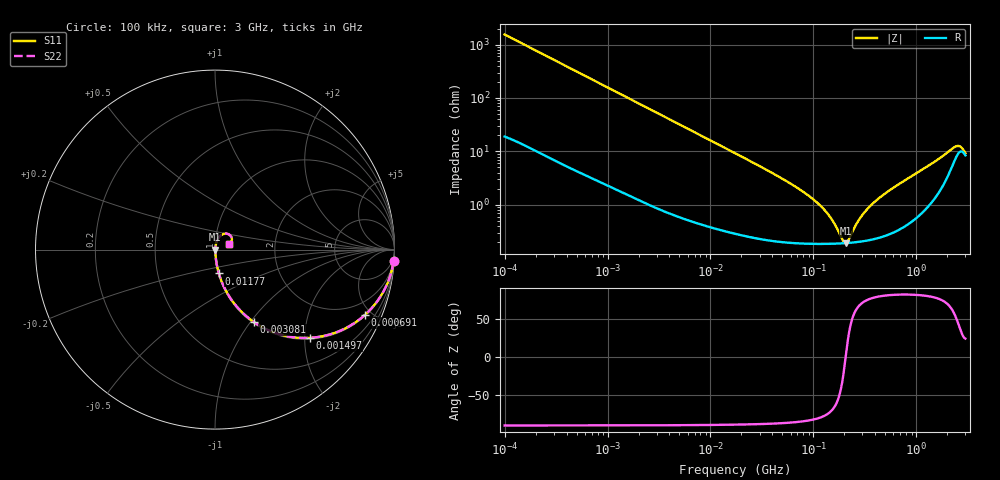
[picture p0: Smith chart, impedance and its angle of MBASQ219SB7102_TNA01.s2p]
! MBASQ219SB7102_TNA01  S-PARAMETER MODEL  ( Standard Model )
! Model Generated by TAIYO YUDEN Corporation (http://www.ty-top.com)
! Version 1.0
! TAIYO YUDEN Control No. 220601
! Copyright(c) 2013 TAIYO YUDEN CO.,LTD. All Rights Reserved.
! Product Description (link to TY-COMPAS)
! https://ds.yuden.co.jp/TYCOMPAS/or/detail?pn=MBASQ219SB7102KTNA01&u=M
! Products Name : Multilayer Ceramic Capacitors
! Characteristics :
!  Capacitance : 1000 [pF] , Rated Voltage : 250 [V] , TCC : X7R
!  Case Size : 2.0 x 1.25 / 0.079 x 0.049 [mm/inch] , Thickness : 0.85 / 0.033 [mm/inch]
!  (Conditions: Temperature = 25 [degC] , DC Bias Voltage = 0 [V])
! External Node Assignments :
!  1  o---| |---o  2
! GND o---------o GND
! Frequency Range : 100kHz  -  3GHz  [ 401 STEP ]
# MHZ S RI R 50
! Freq[MHz].  S11 Real  S11 Imag  S21 Real  S21 Imag  S12 Real  S12 Imag  S22 Real  S22 Imag
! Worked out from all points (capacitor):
!   401 points, 100 kHz to 3 GHz, reference 50 ohm
!   read as one part in series: C = 1.03 nF near 105.3 kHz
!   lowest |Z| = 191 mohm at 205.6 MHz (marker M1)
!   series resonance near 205.7 MHz, so ESL is about 580 pH
!   S11 on the Smith chart (normalised r, x): 100 kHz: 1, -31; 691 kHz: 1.06, -4.55; 1.497 MHz: 1.03, -2.12; 3.081 MHz: 1.02, -1.03; 11.77 MHz: 1.01, -0.27; 3 GHz: 1.17, +0.08
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0.1  0.9951 -0.0643  0.00495 0.0643  0.00495 0.0643  0.9951 -0.0643
0.246461  0.9737 -0.1535  0.0263 0.1535  0.0263 0.1535  0.9737 -0.1535
0.562235  0.883 -0.3146  0.117 0.3146  0.117 0.3146  0.883 -0.3146
0.690972  0.8348 -0.3644  0.1652 0.3644  0.1652 0.3644  0.8348 -0.3644
1.497078  0.5277 -0.4917  0.4723 0.4917  0.4723 0.4917  0.5277 -0.4917
3.080653  0.2149 -0.4027  0.7851 0.4027  0.7851 0.4027  0.2149 -0.4027
3.161081  0.2065 -0.3967  0.7935 0.3967  0.7935 0.3967  0.2065 -0.3967
5.572849  0.0804 -0.2626  0.9196 0.2626  0.9196 0.2626  0.0804 -0.2626
11.76708  0.0216 -0.1331  0.9784 0.1331  0.9784 0.1331  0.0216 -0.1331
17.7727  0.0109 -0.0891  0.9891 0.0891  0.9891 0.0891  0.0109 -0.0891
52.46276  0.00281 -0.0289  0.9972 0.0289  0.9972 0.0289  0.00281 -0.0289
97.38194  0.00202 -0.013  0.998 0.013  0.998 0.013  0.00202 -0.013
139.694  0.00189 -0.00628  0.9981 0.00628  0.9981 0.00628  0.00189 -0.00628
190.323  0.00189 -0.00123  0.9981 0.00123  0.9981 0.00123  0.00189 -0.00123
205.6221  0.00191 -9.02e-06  0.9981 9.02e-06  0.9981 9.02e-06  0.00191 -9.02e-06
216.4987  0.00193 0.000808  0.9981 -0.000808  0.9981 -0.000808  0.00193 0.000808
266.0711  0.00202 0.00412  0.998 -0.00412  0.998 -0.00412  0.00202 0.00412
318.6746  0.00215 0.00717  0.9978 -0.00717  0.9978 -0.00717  0.00215 0.00717
547.5153  0.00312 0.0182  0.9969 -0.0182  0.9969 -0.0182  0.00312 0.0182
2318.426  0.0672 0.0882  0.9328 -0.0882  0.9328 -0.0882  0.0672 0.0882
2637.286  0.0933 0.0646  0.9067 -0.0646  0.9067 -0.0646  0.0933 0.0646
3000  0.079 0.0326  0.921 -0.0326  0.921 -0.0326  0.079 0.0326
